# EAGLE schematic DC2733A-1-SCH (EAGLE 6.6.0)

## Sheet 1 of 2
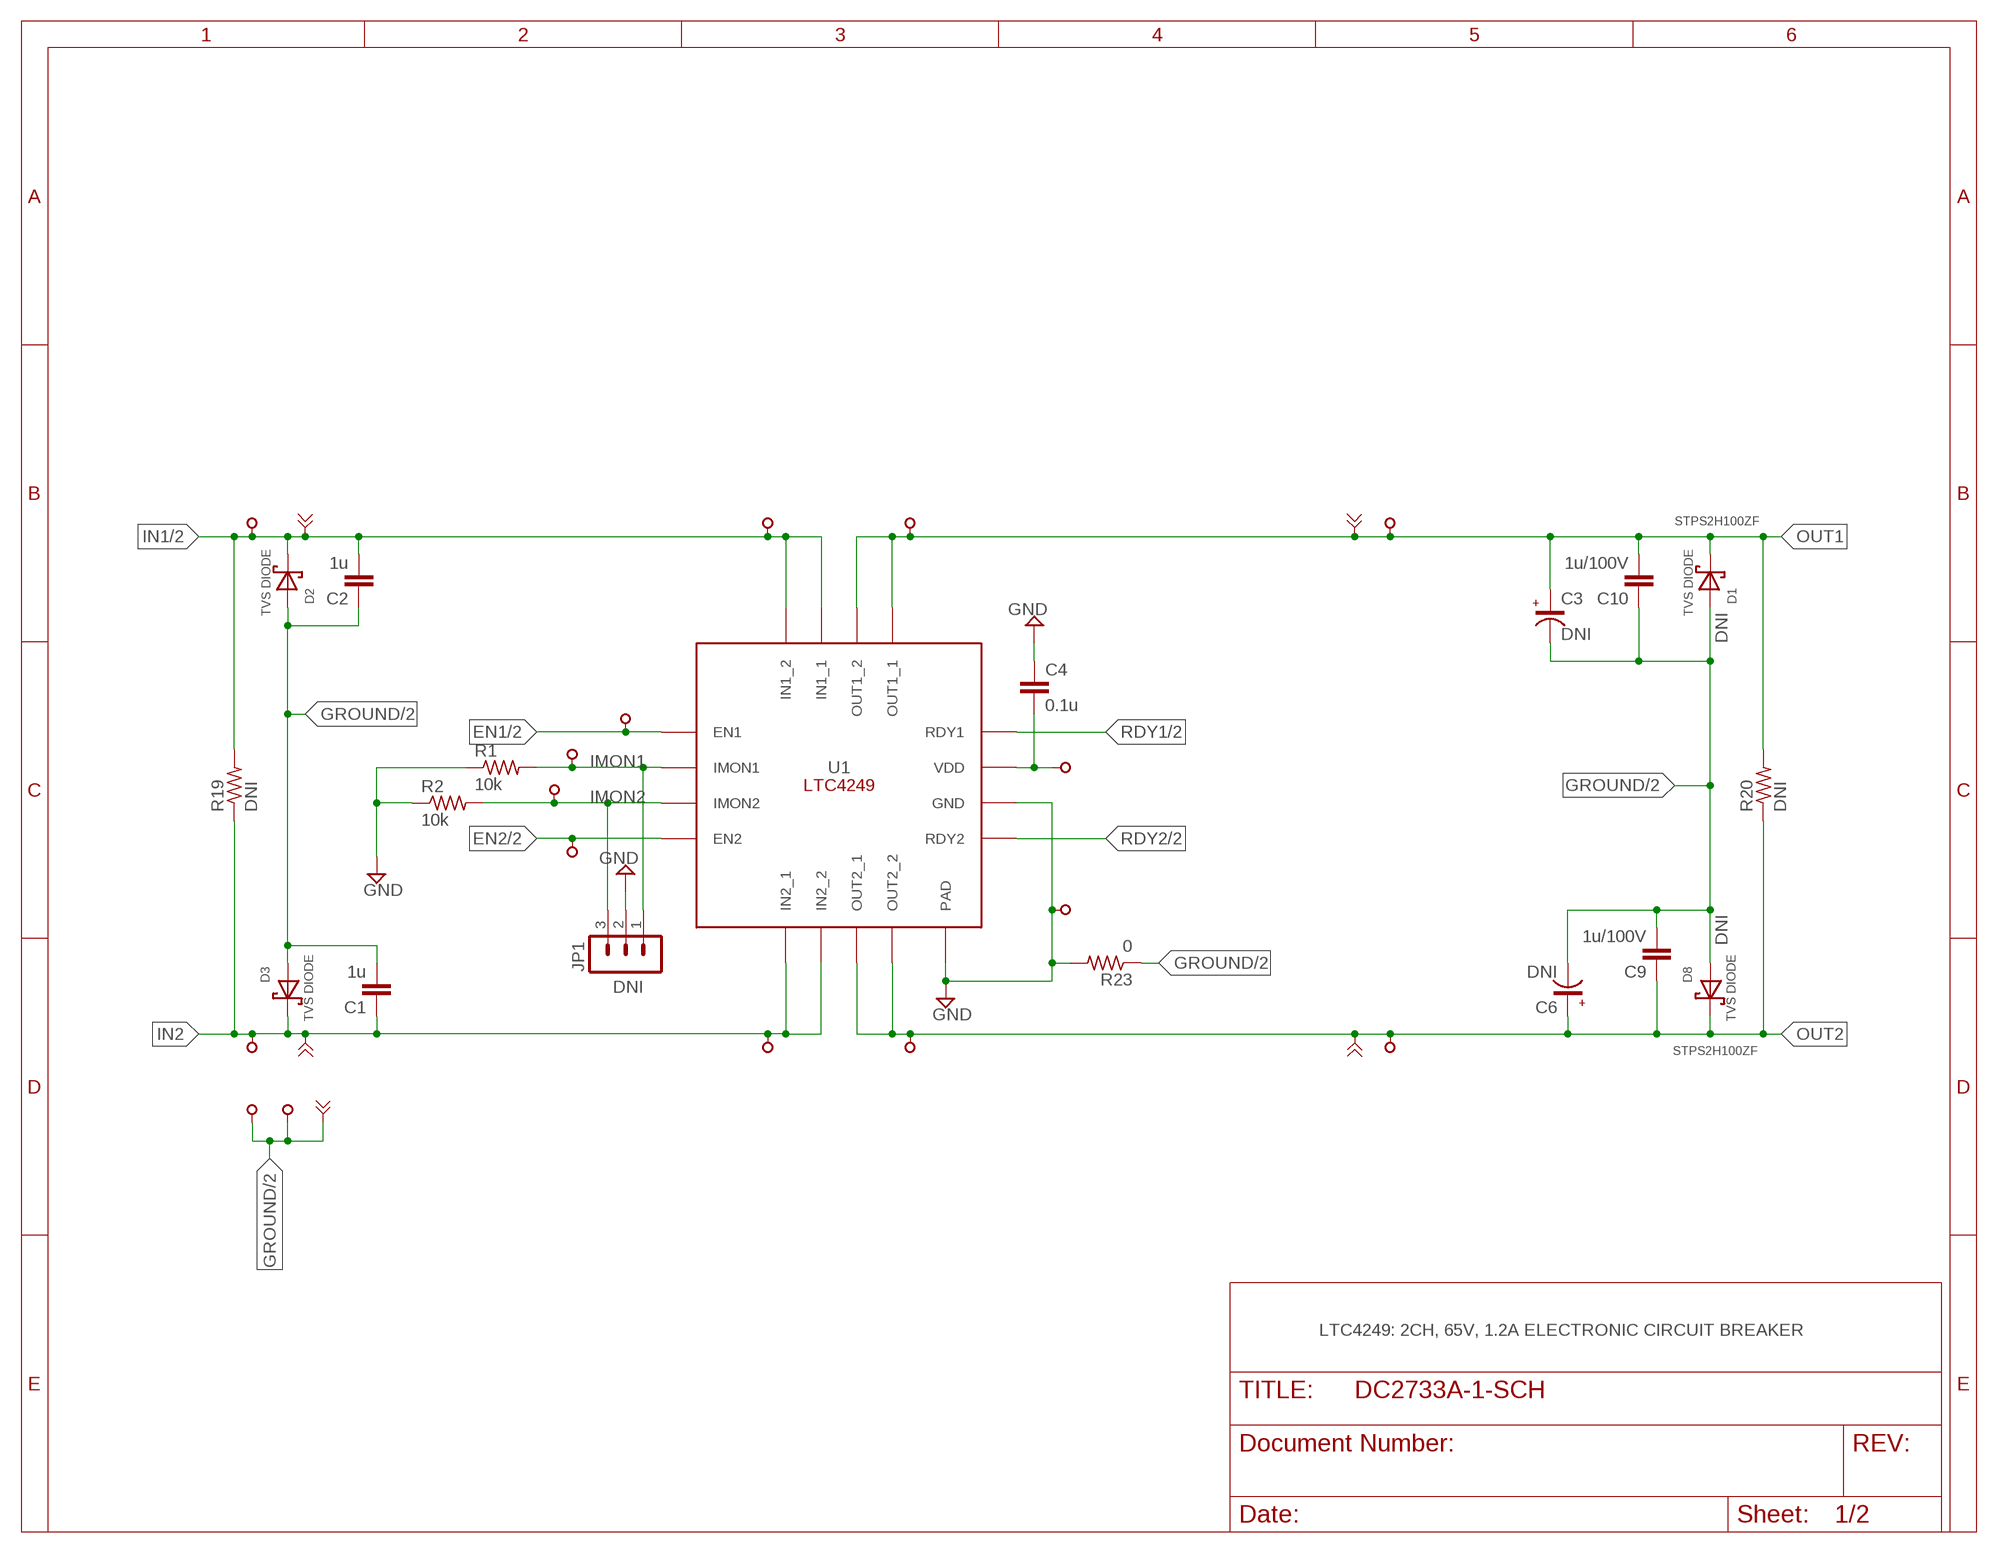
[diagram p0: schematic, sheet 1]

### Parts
C1  1u  CC0805_BOX  [C0805_BOX]
C2  1u  CC0805_BOX  [C0805_BOX]
C3  DNI  CAP  [CAP-CAN]
C4  0.1u  CC0603_BOX  [C0603_BOX]
C6  DNI  CAP  [CAP-CAN]
C9  1u/100V  CC0805_BOX  [C0805_BOX]
C10  1u/100V  CC0805_BOX  [C0805_BOX]
D1  SMCJXXA  [DO-214AB]
D2  SMCJXXA  [DO-214AB]
D3  SMCJXXA  [DO-214AB]
D8  SMCJXXA  [DO-214AB]
J1  BANANA  [BANANA]
J2  BANANA  [BANANA]
J3  BANANA  [BANANA]
J4  BANANA  [BANANA]
J5  BANANA  [BANANA]
JP1  MA03-1  [MA03-1]
R1  10k  RR0402  [R0402_BOX]
R2  10k  RR0402  [R0402_BOX]
R19  DNI  RR1210_BOX  [R1210_BOX]
R20  DNI  RR1210_BOX  [R1210_BOX]
R23  0  RR0402  [R0402_BOX]
TP1  TESTPOINT_BIG  [TP1]
TP2  TESTPOINT_BIG  [TP1]
TP3  TESTPOINT_BIG  [TP1]
TP4  TESTPOINT_BIG  [TP1]
TP6  TESTPOINT_BIG  [TP1]
TP7  TESTPOINT_BIG  [TP1]
TP8  TESTPOINT  [VIA]
TP9  TESTPOINT  [VIA]
TP10  TESTPOINT  [VIA]
TP11  TESTPOINT  [VIA]
TP16  TESTPOINT  [VIA]
TP17  TESTPOINT  [VIA]
TP22  TESTPOINT_BIG  [TP1]
TP23  TESTPOINT_BIG  [TP1]
TP24  TESTPOINT_BIG  [TP1]
TP25  TESTPOINT_BIG  [TP1]
U1  LTC4249-16  [QFN-16-3X3]

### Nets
EN1: TP22.TP U1.P$1(EN1) ; also sheet 2
EN2: TP23.TP U1.P$4(EN2) ; also sheet 2
GND: C4.1 JP1.2 R1.1 R2.1 R23.2 TP17.1 U1.P$10(GND) U1.P$17(PAD)
GROUND: C1.2 C2.1 C3.P$2 C6.P$2 C9.2 C10.1 D1.P$1 D2.P$1 D3.P$1 D8.P$1 J5.1 R23.1 TP6.TP TP7.TP ; also sheet 2
IMON1: JP1.1 R1.2 TP24.TP U1.P$2(IMON1)
IMON2: JP1.3 R2.2 TP25.TP U1.P$3(IMON2)
IN1: C2.2 D2.P$2 J1.1 R19.2 TP1.TP TP8.1 U1.P$15(IN1_1) U1.P$16(IN1_2) ; also sheet 2
IN2: C1.1 D3.P$2 J2.1 R19.1 TP2.TP TP9.1 U1.P$5(IN2_1) U1.P$6(IN2_2)
N$1: C4.2 TP16.1 U1.P$11(VDD)
OUT1: C3.P$1 C10.2 D1.P$2 J4.1 R20.2 TP3.TP TP11.1 U1.P$13(OUT1_1) U1.P$14(OUT1_2)
OUT2: C6.P$1 C9.1 D8.P$2 J3.1 R20.1 TP4.TP TP10.1 U1.P$7(OUT2_1) U1.P$8(OUT2_2)
RDY1: U1.P$12(RDY1) ; also sheet 2
RDY2: U1.P$9(RDY2) ; also sheet 2

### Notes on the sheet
- STPS2H100ZF
- DNI
- DNI
- DNI
- STPS2H100ZF
- LTC4249: 2CH, 65V, 1.2A ELECTRONIC CIRCUIT BREAKER

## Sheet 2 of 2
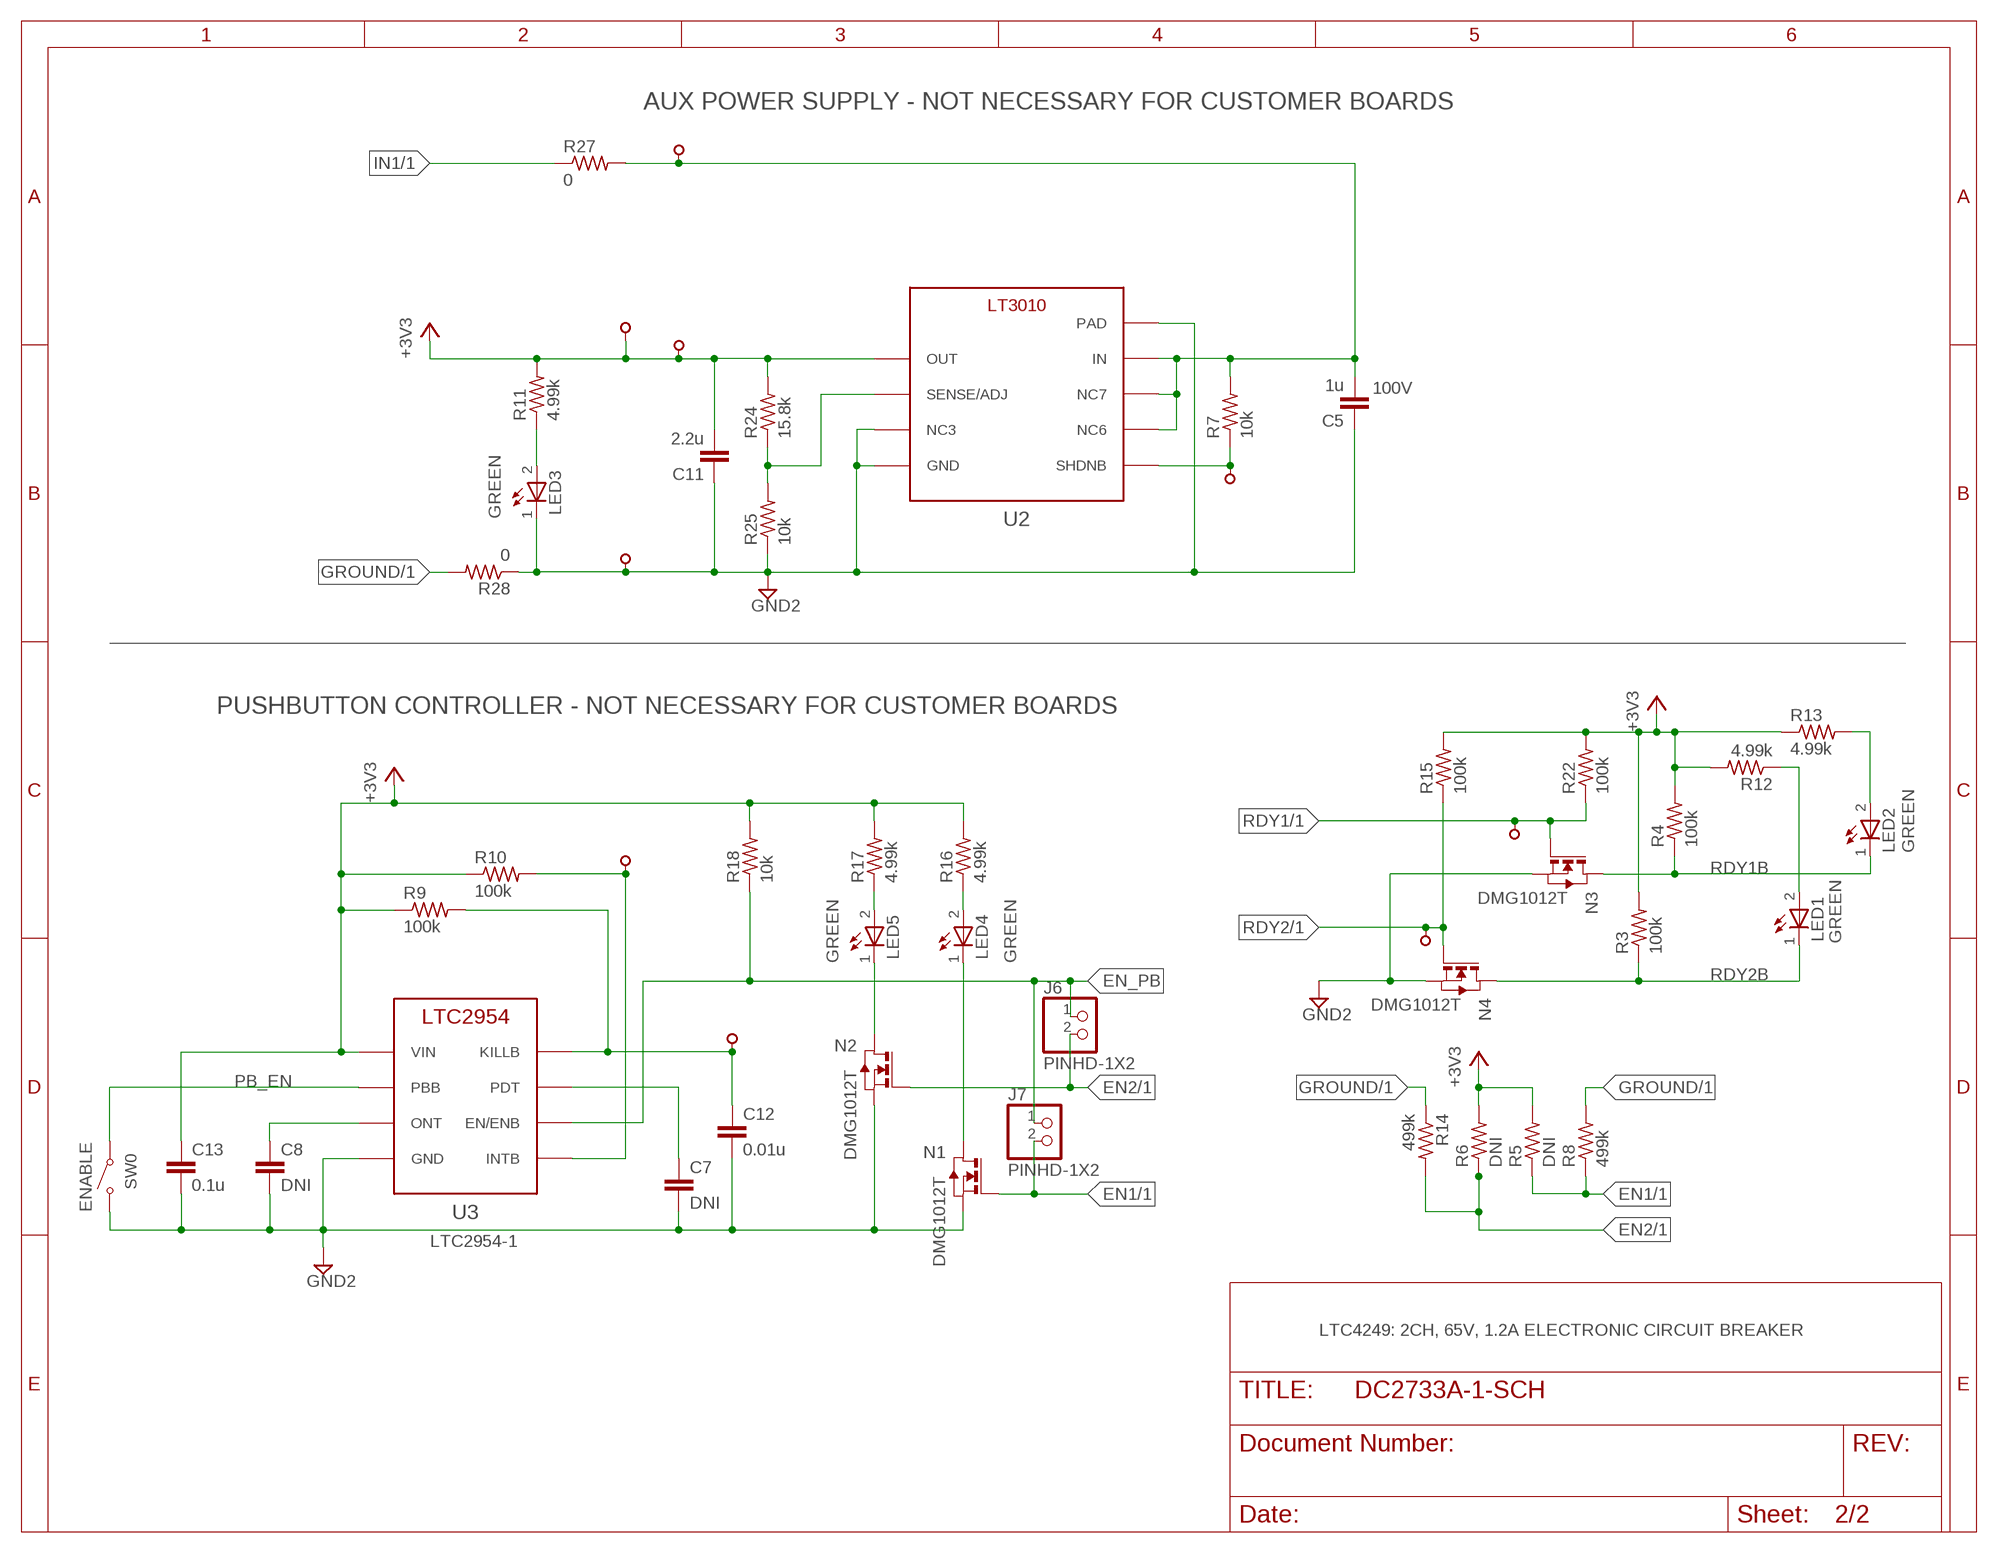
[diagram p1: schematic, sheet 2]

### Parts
C5  1u  CC0805_BOX  [C0805_BOX]
C7  DNI  CC0603_BOX  [C0603_BOX]
C8  DNI  CC0603_BOX  [C0603_BOX]
C11  2.2u  CC0805_BOX  [C0805_BOX]
C12  0.01u  CC0603_BOX  [C0603_BOX]
C13  0.1u  CC0603_BOX  [C0603_BOX]
J6  PINHD-1X2  [1X02]
J7  PINHD-1X2  [1X02]
LED1  LED-0603  [CHIPLED_0603]
LED2  LED-0603  [CHIPLED_0603]
LED3  LED-0603  [CHIPLED_0603]
LED4  LED-0603  [CHIPLED_0603]
LED5  LED-0603  [CHIPLED_0603]
N1  DMG1012T  [SOT523-3]
N2  DMG1012T  [SOT523-3]
N3  DMG1012T  [SOT523-3]
N4  DMG1012T  [SOT523-3]
R3  100k  RR0402  [R0402_BOX]
R4  100k  RR0402  [R0402_BOX]
R5  DNI  RR0402  [R0402_BOX]
R6  DNI  RR0402  [R0402_BOX]
R7  10k  RR0402  [R0402_BOX]
R8  499k  RR0402  [R0402_BOX]
R9  100k  RR0402  [R0402_BOX]
R10  100k  RR0402  [R0402_BOX]
R11  4.99k  RR0402  [R0402_BOX]
R12  4.99k  RR0402  [R0402_BOX]
R13  4.99k  RR0402  [R0402_BOX]
R14  499k  RR0402  [R0402_BOX]
R15  100k  RR0402  [R0402_BOX]
R16  4.99k  RR0402  [R0402_BOX]
R17  4.99k  RR0402  [R0402_BOX]
R18  10k  RR0402  [R0402_BOX]
R22  100k  RR0402  [R0402_BOX]
R24  15.8k  RR0402  [R0402_BOX]
R25  10k  RR0402  [R0402_BOX]
R27  0  RR0402  [R0402_BOX]
R28  0  RR0402  [R0402_BOX]
SW0  PTS635SL25SMTR LFS  SWITCH_PTS635  [SWITCH_PTS635]
TP5  TESTPOINT  [VIA]
TP12  TESTPOINT  [VIA]
TP13  TESTPOINT  [VIA]
TP14  TESTPOINT  [VIA]
TP15  TESTPOINT  [VIA]
TP18  TESTPOINT  [VIA]
TP19  TESTPOINT_BIG  [TP1]
TP20  TESTPOINT_BIG  [TP1]
TP21  TESTPOINT_BIG  [TP1]
U2  LT3010  [MS8E]
U3  LTC2954  [TSOT23-8]

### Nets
+3V3: C11.2 C13.1 R3.2 R4.2 R5.2 R6.2 R9.1 R10.1 R11.2 R12.2 R13.1 R15.2 R16.2 R17.2 R18.2 R22.2 R24.2 TP12.1 TP19.TP U2.P$1(OUT) U3.P1(VIN)
EN1: J7.2 N1.G R5.1 R8.1 ; also sheet 1
EN2: J6.2 N2.G R6.1 R14.2 ; also sheet 1
EN_PB: J6.1 J7.1 R18.1 U3.P6(EN/ENB)
GND2: C5.1 C7.2 C8.2 C11.1 C12.2 C13.2 LED3.C N1.S N2.S N3.S N4.S R25.1 R28.1 SW0.SW1 TP13.1 U2.P$3(NC3) U2.P$4(GND) U2.P$9(PAD) U3.P4(GND)
GROUND: R8.2 R14.1 R28.2 ; also sheet 1
IN1: R27.1 ; also sheet 1
N$2: LED2.A R13.2
N$3: LED1.A R12.1
N$4: C8.1 U3.P3(ONT)
N$5: C7.1 U3.P7(PDT)
N$6: LED3.A R11.1
N$7: LED5.C N2.D
N$8: C12.1 R9.2 TP18.1 U3.P8(KILLB)
N$9: LED4.C N1.D
N$10: R24.1 R25.2 U2.P$2(SENSE/ADJ)
N$11: R10.2 TP15.1 U3.P5(INTB)
N$12: LED4.A R16.1
N$13: R7.1 TP5.1 U2.P$5(SHDNB)
N$14: LED5.A R17.1
PB_EN: SW0.SW2 U3.P2(PBB)
RDY1: N3.G R22.1 TP20.TP ; also sheet 1
RDY1B: LED2.C N3.D R4.1
RDY2: N4.G R15.1 TP21.TP ; also sheet 1
RDY2B: LED1.C N4.D R3.1
V1: C5.2 R7.2 R27.2 TP14.1 U2.P$6(NC6) U2.P$7(NC7) U2.P$8(IN)

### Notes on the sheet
- AUX POWER SUPPLY - NOT NECESSARY FOR CUSTOMER BOARDS
- 100V
- GREEN
- PUSHBUTTON CONTROLLER - NOT NECESSARY FOR CUSTOMER BOARDS
- GREEN
- GREEN
- GREEN | GREEN
- ENABLE
- LTC2954-1
- LTC4249: 2CH, 65V, 1.2A ELECTRONIC CIRCUIT BREAKER

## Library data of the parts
C1 C2 C4 C5 C7-C13 = kalin:C: CAPACITOR, European symbol
C3 C6 = nengerLib:CAP: CAPACITOR, European symbol
D1-D3 D8 = nengerLib:SMCJXXA: TVS DIODE BOURNS SMCJXXA
J1-J5 = kalin:BANANA: Banana connector
J6 J7 = nengerLib:PINHD-1X2: PINHEADER 1x3 2mm
JP1 = con-lstb:MA03-1: PIN HEADER; OC_FARNELL: unknown; OC_NEWARK: unknown
LED1-LED5 = kalin:LED-0603: SMD LED in R0603
N1-N4 = nengerLib:DMG1012T: Diodes Inc. N-Channel Enhancement Mode N-MOSFET
R1-R20 R22-R25 R27 R28 = kalin:R: RESISTOR, American symbol
SW0 = kalin:SWITCH_PTS635: PTS635SL25 Surface Mount Tactile Switch
TP1-TP4 TP6 TP7 TP19-TP25 = kalin:TESTPOINT_BIG: Large Test Point
TP5 TP8-TP18 = kalin:TESTPOINT: Test Point
U1 = LTC-DEVICES:LTC4249-16: LTC4249 65V, 75 mΩ R ON Dual Electronic Circuit Breaker
U2 = LTC-DEVICES:LT3010: 50mA, 3V to 80V Low Dropout Micropower Linear Regulator
U3 = LTC-DEVICES:LTC2954: Pushbutton On/Off Controller with μP Interrupt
